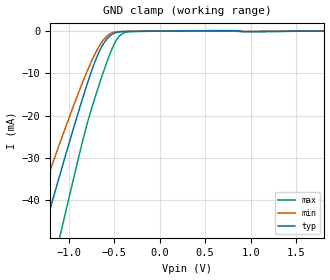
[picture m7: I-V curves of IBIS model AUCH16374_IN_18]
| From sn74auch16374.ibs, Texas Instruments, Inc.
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[Model]   AUCH16374_IN_18
Model_type  Input
Vinl=0.5775
Vinh=1.2675
| variable   typ   min   max
C_comp   2.73pF   2.14pF   3.16pF
[Temperature Range]   40   100   -40
| Ambient temperature   25   85   -40
[Voltage range]   1.8   1.65   1.95
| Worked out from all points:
|   GND clamp passes 1 mA (typ) near -0.54 V on its own axis
[GND Clamp]
| AUCH16374_IN_18
|   Voltage   I(typ)   I(min)   I(max)
-3.6V     -229mA     -190.7mA   -276.9mA
-1.43V    -59.59mA   -47.26mA   -79.59mA
-1.295V   -49.21mA   -38.78mA   -67.14mA
-1.255V   -46.16mA   -36.29mA   -63.45mA
-1.1V     -34.43mA   -26.81mA   -49.16mA
-1.05V    -30.7mA    -23.82mA   -44.56mA
-815mV    -13.85mA   -10.51mA   -23.48mA
-680mV    -5.661mA   -4.2mA     -13.77mA
-560mV    -1.419mA   -836.5uA   -6.202mA
-485mV    -387.3uA   -198.7uA   -2.536mA
-420mV    -131uA     -73.74uA   -760.5uA
1.8V      232pA      557.8nA    -933.9pA
